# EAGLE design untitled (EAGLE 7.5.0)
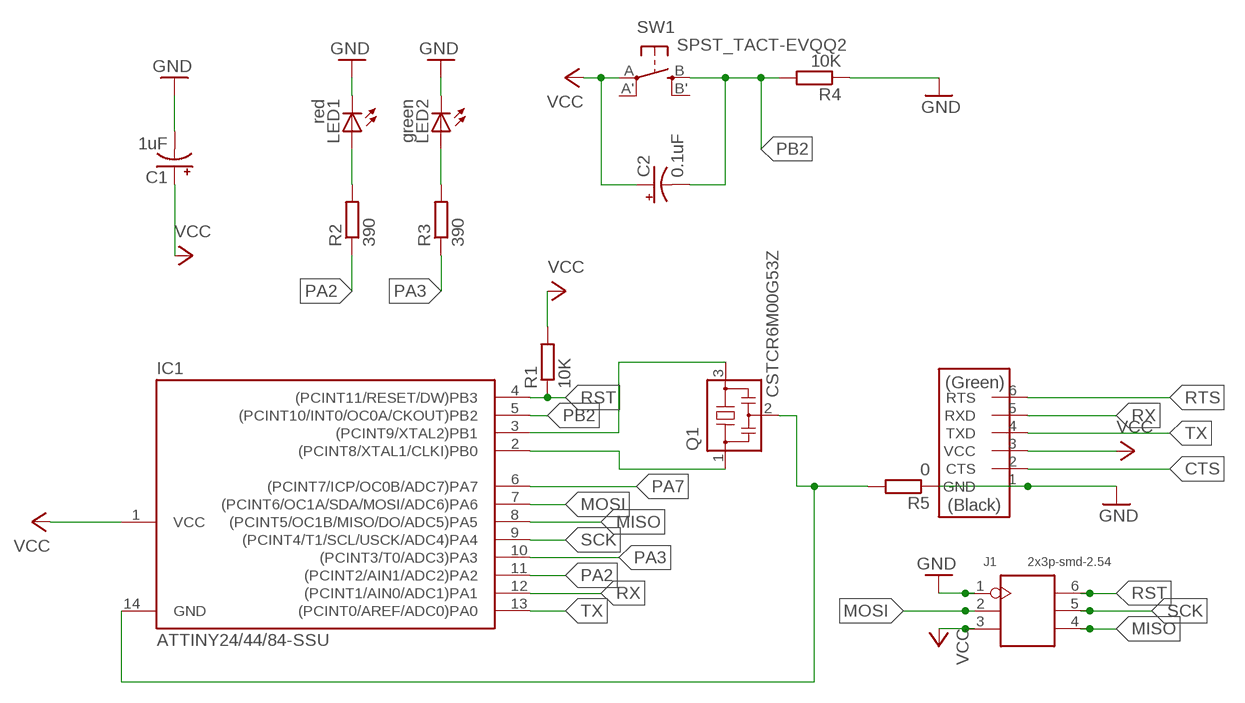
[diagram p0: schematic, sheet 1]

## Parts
C1  1uF  CAP_POL1206-KIT  [EIA3216-KIT]
C2  0.1uF  CAP_POL1206-KIT  [EIA3216-KIT]
IC1  ATTINY24/44/84-SSU  [SOIC14]
J1  2x3p-smd-2.54  SMD-BLUE-FEMALE-HEADER-VERT(2X3P-2.54)  [H2X3-SMD-2.54]
LED1  red  LEDP-LCC-2  [P-LCC-2]
LED2  green  LEDP-LCC-2  [P-LCC-2]
Q1  CSTCR6M00G53Z  [CSTCR6M]
R1  10K  R-EU_M1206  [M1206]
R2  390  R-EU_M1206  [M1206]
R3  390  R-EU_M1206  [M1206]
R4  10K  R-EU_M1206  [M1206]
R5  0  R-EU_M1206  [M1206]
SW1  SPST_TACT-EVQQ2  [EVQ-Q2]
U$1  FTDI-SMD-HEADER  [1X06SMD]

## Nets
CTS: U$1.2(CTS)
GND: C1.C(-) J1.1 LED1.C LED2.C R4.1 R5.1 U$1.1(GND)
MISO: IC1.8((PCINT5/OC1B/MISO/DO/ADC5)PA5) J1.4
MOSI: IC1.7((PCINT6/OC1A/SDA/MOSI/ADC6)PA6) J1.2
N$1: IC1.2((PCINT8/XTAL1/CLKI)PB0) Q1.1
N$4: LED1.A R2.2
N$5: IC1.14(GND) Q1.2 R5.2
N$11: LED2.A R3.2
PA2: IC1.11((PCINT2/AIN1/ADC2)PA2) R2.1
PA3: IC1.10((PCINT3/T0/ADC3)PA3) R3.1
PA7: IC1.6((PCINT7/ICP/OC0B/ADC7)PA7)
PB1: IC1.3((PCINT9/XTAL2)PB1) Q1.3
PB2: C2.C(-) IC1.5((PCINT10/INT0/OC0A/CKOUT)PB2) R4.2 SW1.B(S)
RST: IC1.4((PCINT11/RESET/DW)PB3) J1.6 R1.1
RTS: U$1.6(RTS)
RX: IC1.12((PCINT1/AIN0/ADC1)PA1) U$1.5(RXD)
SCK: IC1.9((PCINT4/T1/SCL/USCK/ADC4)PA4) J1.5
TX: IC1.13((PCINT0/AREF/ADC0)PA0) U$1.4(TXD)
VCC: C1.A(+) C2.A(+) IC1.1(VCC) J1.3 R1.2 SW1.A(P) U$1.3(VCC)
Unconnected: SW1.A'(P1) SW1.B'(S1)

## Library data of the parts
C1 C2 = SparkFun-Passives:CAP_POL: Capacitor Polarized
IC1 = attiny24_44_84:ATTINY24/44/84
J1 = Seeed-OPL-Connector:SMD-BLUE-FEMALE-HEADER-VERT(2X3P-2.54): 320030035; MPN: F185-1203A1BMYA1
LED1 LED2 = adafruit:LED: LED
Q1 = murata-filter:CSTCR: Resonator Source: murata.co.jp; MPN: CSTCR6M00G53-R0; OC_FARNELL: 1170434; OC_NEWARK: 25M8759
R1-R5 = rcl:R-EU_: RESISTOR, European symbol
SW1 = adafruit:SPST_TACT: SMT 6mm switch, EVQQ2 series http://www.ladyada.net/library/eagle
U$1 = fab:FTDI-SMD-HEADER

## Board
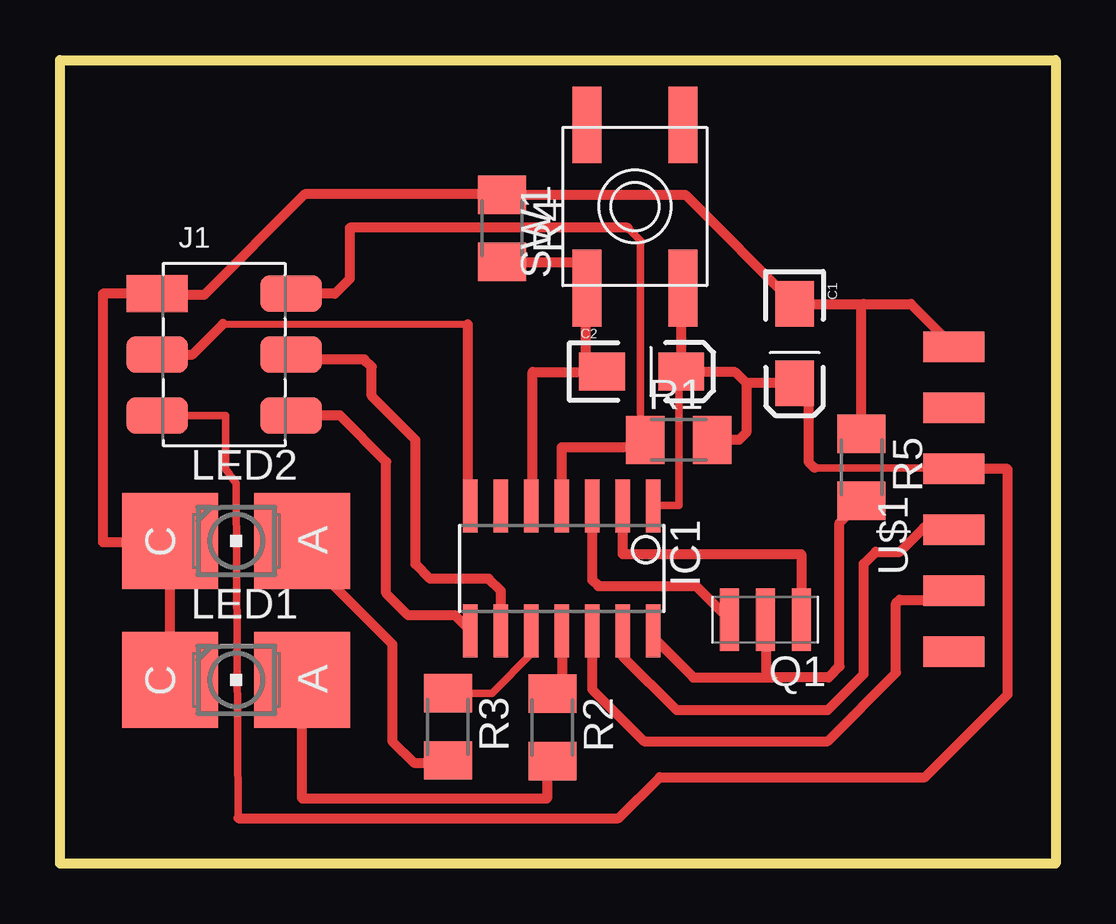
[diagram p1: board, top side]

Size 41.5 x 33.5 mm. Coordinates in mm from the lower left corner, seen from the top.
Outline: 0,0 41.5,0 41.5,33.5 0,33.5 0,0
Copper layers (1*16): Top 0.035mm / dielectric 1.5mm / Bottom 0.035mm
Design rules "default *": minimum track width 10mil, minimum drill 24mil, track to track 12mil, track to pad 12mil, pad to pad 13mil, via to via 13mil, smd to smd 13mil, copper to edge 40mil, drill to drill 8mil, minimum pad ring 10mil, minimum via ring 8mil, stop-mask expansion 4mil, vias tented up to drill 0mil, thermal gap 10mil
Milling: 4 lines

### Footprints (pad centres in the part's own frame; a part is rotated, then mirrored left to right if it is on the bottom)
EIA3216-KIT = smd 1.9 x 1.6: A 1.65,0; C -1.65,0
SOIC14 = smd 0.61 x 2.21: 1 -3.81,-2.603; 2 -2.54,-2.603; 3 -1.27,-2.603; 4 0,-2.603; 5 1.27,-2.603; 6 2.54,-2.603; 7 3.81,-2.603; 8 3.81,2.603; 9 2.54,2.603; 10 1.27,2.603; 11 0,2.603; 12 -1.27,2.603; 13 -2.54,2.603; 14 -3.81,2.603
H2X3-SMD-2.54 = smd 2.54 x 1.524: 1 -2.794,2.54; 2 -2.794,0; 3 -2.794,-2.54; 4 2.794,-2.54; 5 2.794,0; 6 2.794,2.54
P-LCC-2 = smd 4 x 4: A 0,2.75; C 0,-2.75
CSTCR6M = smd 0.8 x 2.6: 1 -1.5,0; 2 0,0; 3 1.5,0
M1206 = smd 1.6 x 2: 1 -1.4,0; 2 1.4,0
EVQ-Q2 = smd 3.2 x 1.2: A -3.4,-2; A' 3.4,-2; B -3.4,2; B' 3.4,2
1X06SMD = smd 2.54 x 1.27: 1 0,6.35; 2 0,3.81; 3 0,1.27; 4 0,-1.27; 5 0,-3.81; 6 0,-6.35

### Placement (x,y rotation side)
C1  30.62,21.68 270 top
C2  24.24,20.51 0 top
IC1  20.92,12.3 180 top
J1  6.85,21.22 0 top
LED1  7.35,7.66 270 top
LED2  7.35,13.45 270 top
Q1  29.4,10.17 180 top
R1  25.79,17.66 0 top
R2  20.52,5.68 270 top
R3  16.17,5.7 270 top
R4  18.43,26.48 270 top
R5  33.41,16.52 270 top
SW1  23.96,27.39 90 top
U$1  37.26,15.19 0 top

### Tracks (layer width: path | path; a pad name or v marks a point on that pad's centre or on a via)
GND
  Top 0.406: LED1.C LED2.C 4.6,13.4 1.79,13.4 1.79,23.76 J1.1 | 3.85,23.96 J1.1 | 33.5,23.33 C1.C 26.07,27.88 R4.1 18.4,27.9 10.2,27.9 6,23.7 4.11,23.7 J1.1 | 33.5,23.33 35.47,23.33 U$1.1 | R5.1 33.41,23.24 33.5,23.33
MISO
  Top 0.406: IC1.8 16.46,10.35 14.52,10.35 13.6,11.26 13.6,16.75 11.67,18.68 J1.4
MOSI
  Top 0.29: 17,22.48 6.8,22.48
  Top 0.3: IC1.7 17,14.91 | 6.8,22.48 6.8,22.49
  Top 0.406: J1.2 5.53,21.22 6.8,22.49 | 17,14.91 17,22.48
N$1
  Top 0.406: IC1.2 23.45,12.9 30.9,12.9 Q1.1
N$4
  Top 0.406: 11.16,7.66 LED1.A 10.1,2.7 20.3,2.7 20.3,4.28 R2.2
N$5  (1 unrouted)
  Top 0.406: IC1.14 24.73,9.28 24.88,9.28 26.4,7.76 29.68,7.76 | 29.91,7.76 29.98,7.68 | 29.68,7.76 32.04,7.76 32.5,8.21 32.5,14.21 R5.2 | 29.68,7.76 29.45,7.99 29.45,10.12 Q1.2
N$11
  Top 0.406: LED2.A 10.1,12.9 13.85,9.15 13.85,5.1 14.75,4.2 16.07,4.2 R3.2
PA2
  Top 0.406: IC1.11 20.92,7.62 R2.1
PA3
  Top 0.305: IC1.10 19.7,9.65 19.7,8.8 18,7.1 R3.1
PB1
  Top 0.406: Q1.3 26.5,11.57 22.44,11.57 22.19,11.82 IC1.3
PB2
  Top 0.406: IC1.5 19.7,14.96 19.7,20.5 21.9,20.5 | 21.9,20.5 C2.C | 21.9,20.5 21.9,23.99 SW1.B 21.96,25.08 R4.2
RST
  Top 0.305: 23.66,26.5 24.24,25.92 24.19,25.92 24.19,18.27 24.39,18.27 R1.1
  Top 0.406: IC1.4 20.92,17.36 24.24,17.36 R1.1 | 23.66,26.5 12.08,26.5 12.08,24.37 11.47,23.76 J1.6
RX
  Top 0.406: IC1.12 22.19,7.26 24.35,5.1 32,5.1 34.85,7.95 34.85,10.85 35,11 36.88,11 U$1.5
SCK
  Top 0.406: IC1.9 18.38,11.37 17.87,11.87 15.43,11.87 14.82,12.48 14.82,17.66 12.99,19.49 12.99,20.71 12.69,21.02 9.84,21.02 J1.5
TX
  Top 0.406: IC1.13 23.46,8.64 25.7,6.4 32,6.4 33.5,7.9 33.5,12.5 34,13 35,13 36,14 37.18,14 U$1.4
VCC
  Top 0.305: C2.A 25.79,20.51 25.79,14.92 IC1.1 | 7.43,1.89 7.35,15.84 6.9,16.45 6.9,18.68 J1.3 | 31.46,16.5 37.26,16.5 U$1.3
  Top 0.406: SW1.A 25.89,23.99 | C1.A | C1.A 28.61,20.03 | 28.61,20.03 28.16,20.48 25.92,20.48 C2.A 25.89,23.99 | 28.61,20.03 28.61,17.97 28.31,17.66 R1.2 | C1.A 31.2,19.44 31.2,16.75 31.46,16.5 | 7.43,1.89 23.29,1.89 25,3.6 36.06,3.6 39.51,7.05 39.51,16.45 37.26,16.45 U$1.3 | 25.67,23.99 25.89,23.99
